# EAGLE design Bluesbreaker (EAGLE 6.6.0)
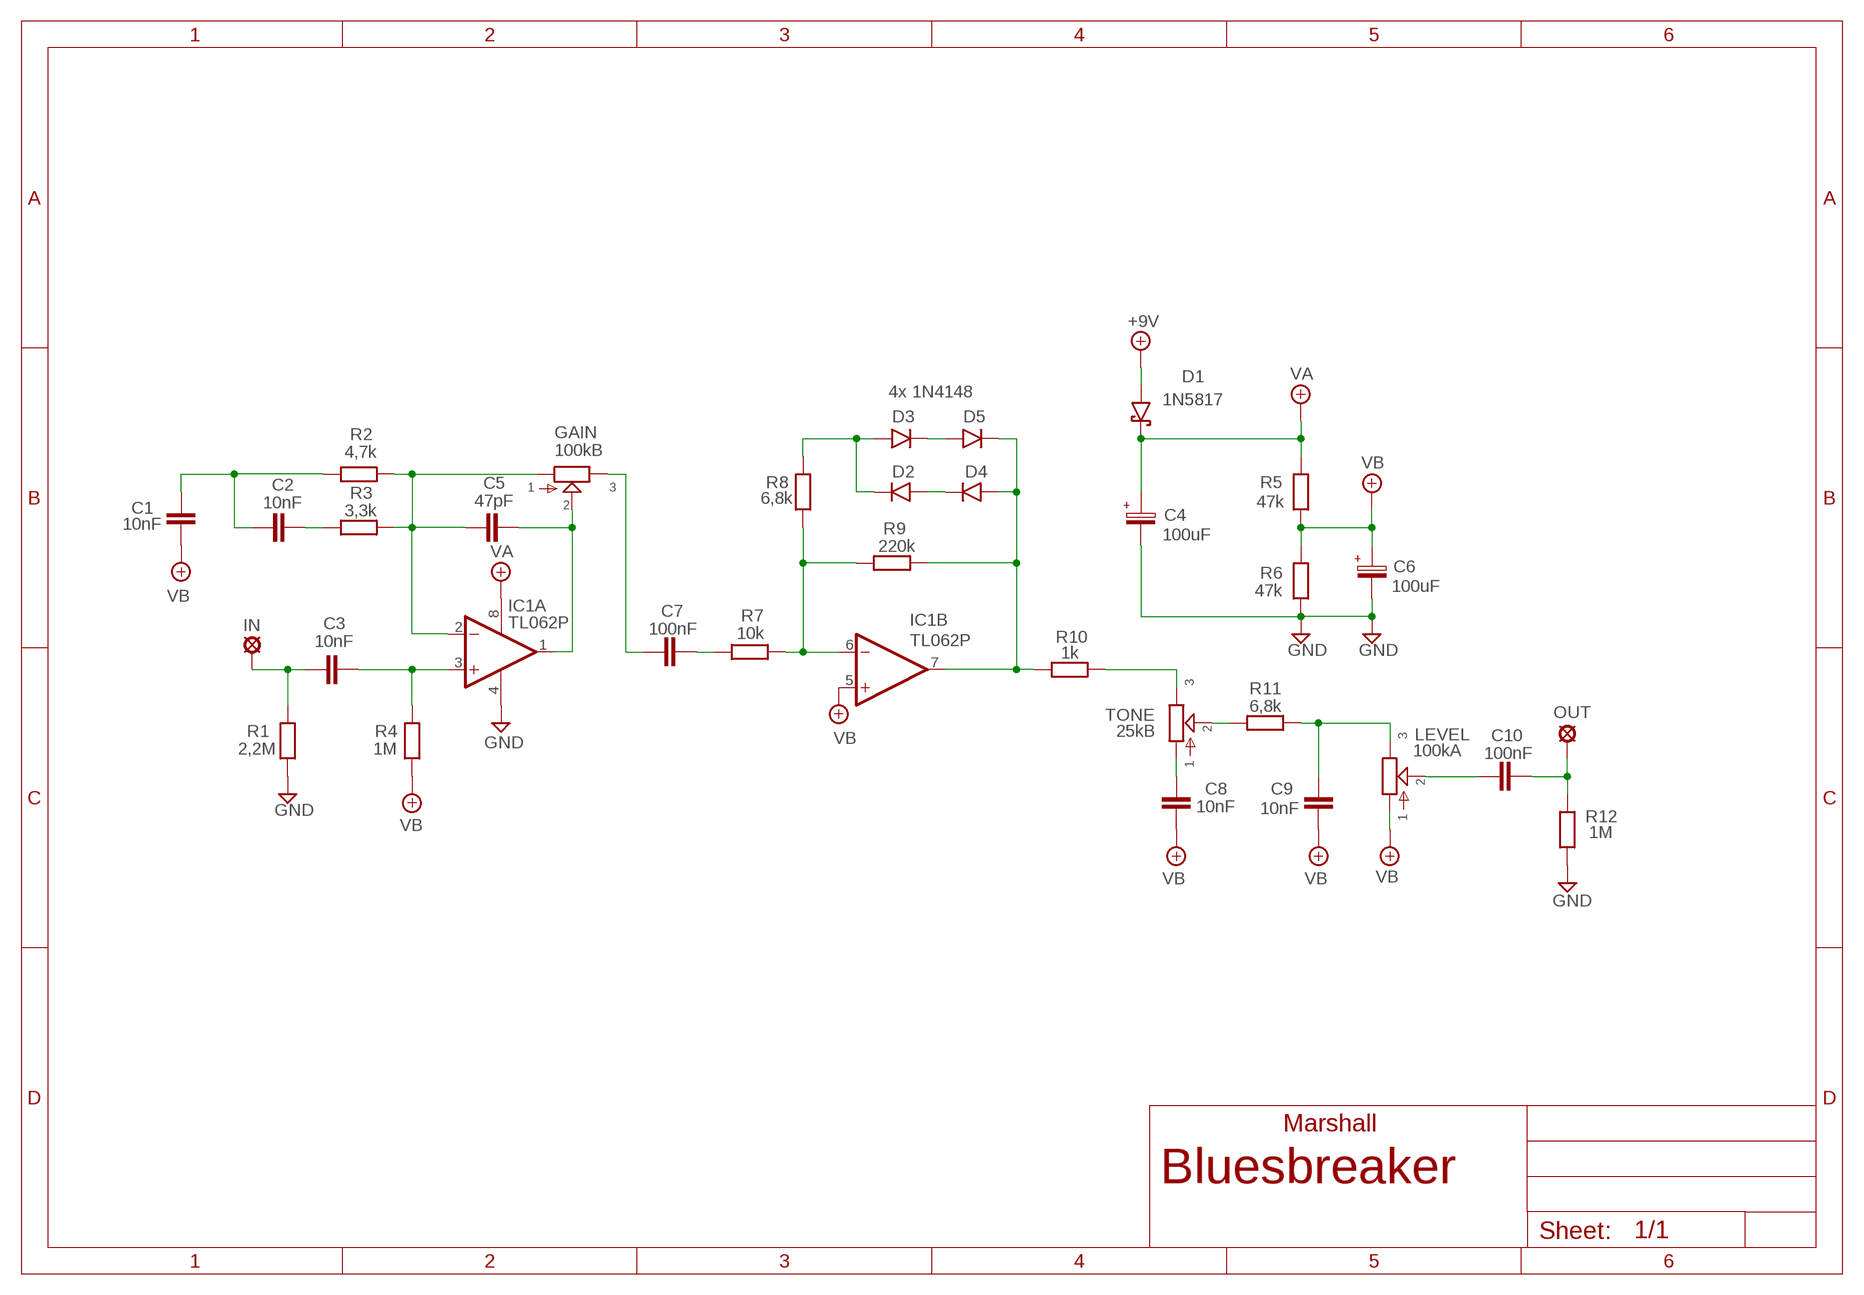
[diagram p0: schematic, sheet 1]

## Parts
+9V  +9V  +9V(T)1  [ROUND]
C1  10nF  1NF-15NF  [3,5MM]
C2  10nF  1NF-15NF  [3,5MM]
C3  10nF  1NF-15NF  [3,5MM]
C4  100uF  063-EU  [063_025]
C5  47pF  050X030_0251  [050X030_025]
C6  100uF  063-EU  [063_025]
C7  100nF  100NF-220NF  [7,5MM]
C8  10nF  1NF-15NF  [3,5MM]
C9  10nF  1NF-15NF  [3,5MM]
C10  100nF  100NF-220NF  [7,5MM]
D1  1N5817  [DO41-3]
D2  1N4148-3  [DO35-3]
D3  4x 1N4148  1N4148-3  [DO35-3]
D4  1N4148-3  [DO35-3]
D5  1N4148-3  [DO35-3]
GAIN  100kB  POT-EU16MM  [16MM]
GND  GND  GND(T)1  [ROUND]
GND5  GND  GND(T)1  [ROUND]
IC1  TL062P  [DIL08]
IN  MCS10B  [MCS10B]
LEVEL  100kA  POT-EU16MM  [16MM]
OUT  MCS10B  [MCS10B]
R1  2,2M  6MM-EU3  [R0207/3]
R2  4,7k  6MM-EU3  [R0207/3]
R3  3,3k  6MM-EU3  [R0207/3]
R4  1M  6MM-EU3  [R0207/3]
R5  47k  6MM-EU3  [R0207/3]
R6  47k  6MM-EU3  [R0207/3]
R7  10k  6MM-EU3  [R0207/3]
R8  6,8k  6MM-EU3  [R0207/3]
R9  220k  6MM-EU3  [R0207/3]
R10  1k  6MM-EU3  [R0207/3]
R11  6,8k  6MM-EU3  [R0207/3]
R12  1M  6MM-EU3  [R0207/3]
TONE  25kB  POT-EU16MM  [16MM]

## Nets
+9V: +9V.1(+9V) D1.A
GND: C4.- C6.- GND5.1(GND) GND.1(GND) IC1.4(P:V-) R1.1 R6.1 R12.2
N$1: C3.2 IN.MP R1.2
N$2: C7.P$1 GAIN.3
N$3: C7.P$2 R7.2
N$4: C3.1 IC1.3(A:+IN) R4.2
N$5: C5.1 GAIN.1 IC1.2(A:-IN) R2.1 R3.1
N$6: C5.2 GAIN.2 IC1.1(A:OUT)
N$7: IC1.6(B:-IN) R7.1 R8.2 R9.2
N$8: C1.1 C2.2 R2.2
N$9: C2.1 R3.2
N$10: R10.1 TONE.3
N$11: D3.C D5.A
N$12: D4.A D5.C IC1.7(B:OUT) R9.1 R10.2
N$13: D2.A D4.C
N$14: C8.1 TONE.1
N$15: D2.C D3.A R8.1
N$16: R11.2 TONE.2
N$17: C9.1 LEVEL.3 R11.1
N$18: C10.P$1 LEVEL.2
N$19: C10.P$2 OUT.MP R12.1
VA: C4.+ D1.C IC1.8(P:V+) R5.2
VB: C1.2 C6.+ C8.2 C9.2 IC1.5(B:+IN) LEVEL.1 R4.1 R5.1 R6.2

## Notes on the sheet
- Marshall

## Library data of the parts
+9V = gm-supply:+9V(T): +9V Voltage Supply
C1-C3 C8 C9 = Mylar Kondensaattorit:1NF-15NF: 1nF-15nF
C4 C6 = Elektrolyytit:063-EU
C5 = Keraamiset kondensaattorit:050X030_025: 47 - 120pF
C7 C10 = Mylar Kondensaattorit:100NF-220NF: 100nF-220nF
D1 = Diodit:1N5817
D2-D5 = Diodit:1N4148: Fast Switching Diode
GAIN LEVEL TONE = gm-pots:POT-EU
GND GND5 = gm-supply:GND(T): Ground
IC1 = Operaatiovahvistimet:TL062: OP AMP
IN OUT = Padit:MCS10B: SOLDER PAD
R1-R12 = Vastukset:6MM-EU: 6mm Resistors (European schematic symbol)

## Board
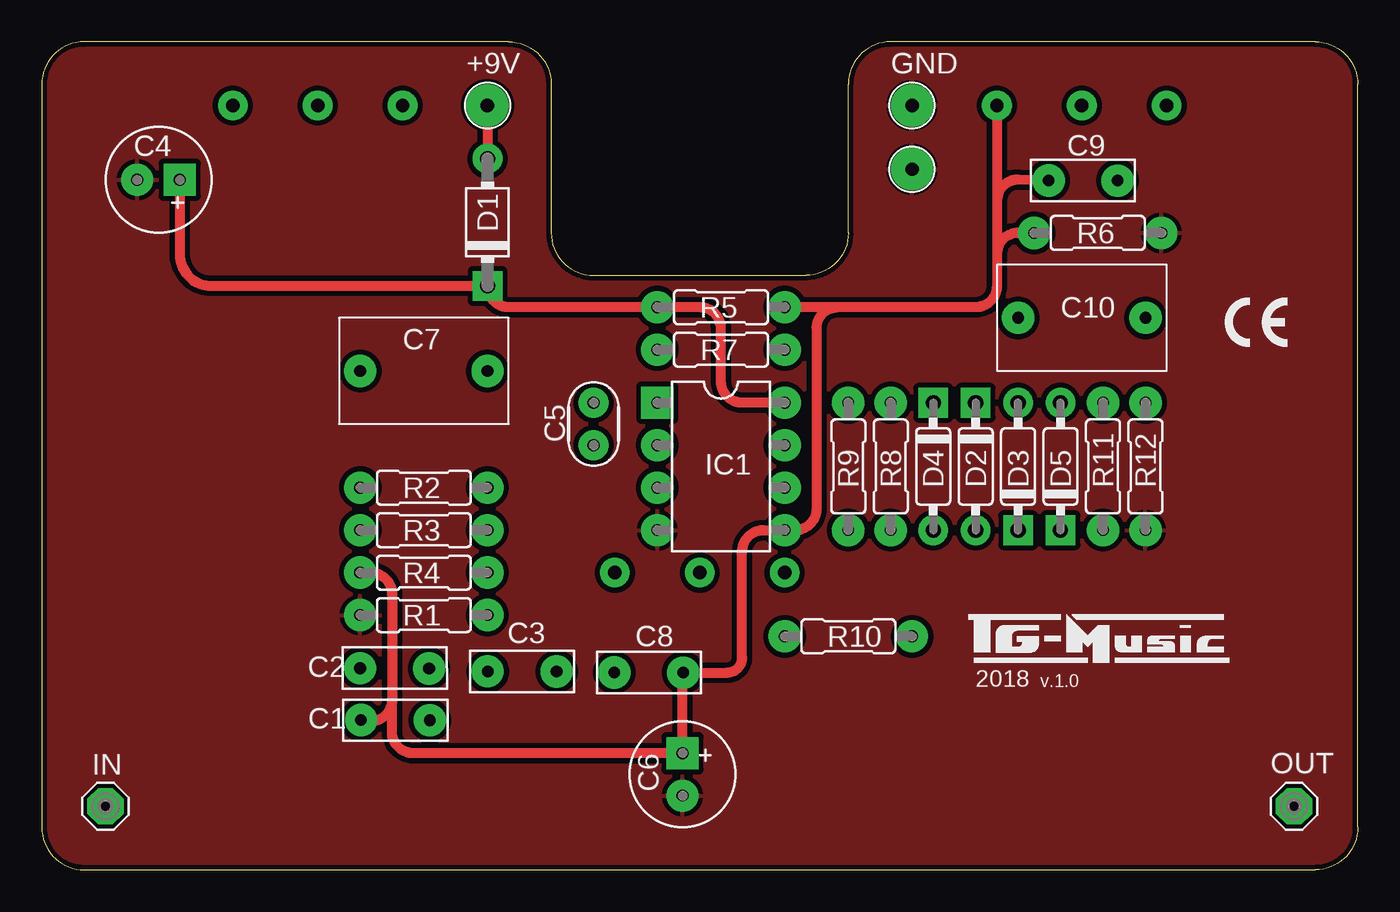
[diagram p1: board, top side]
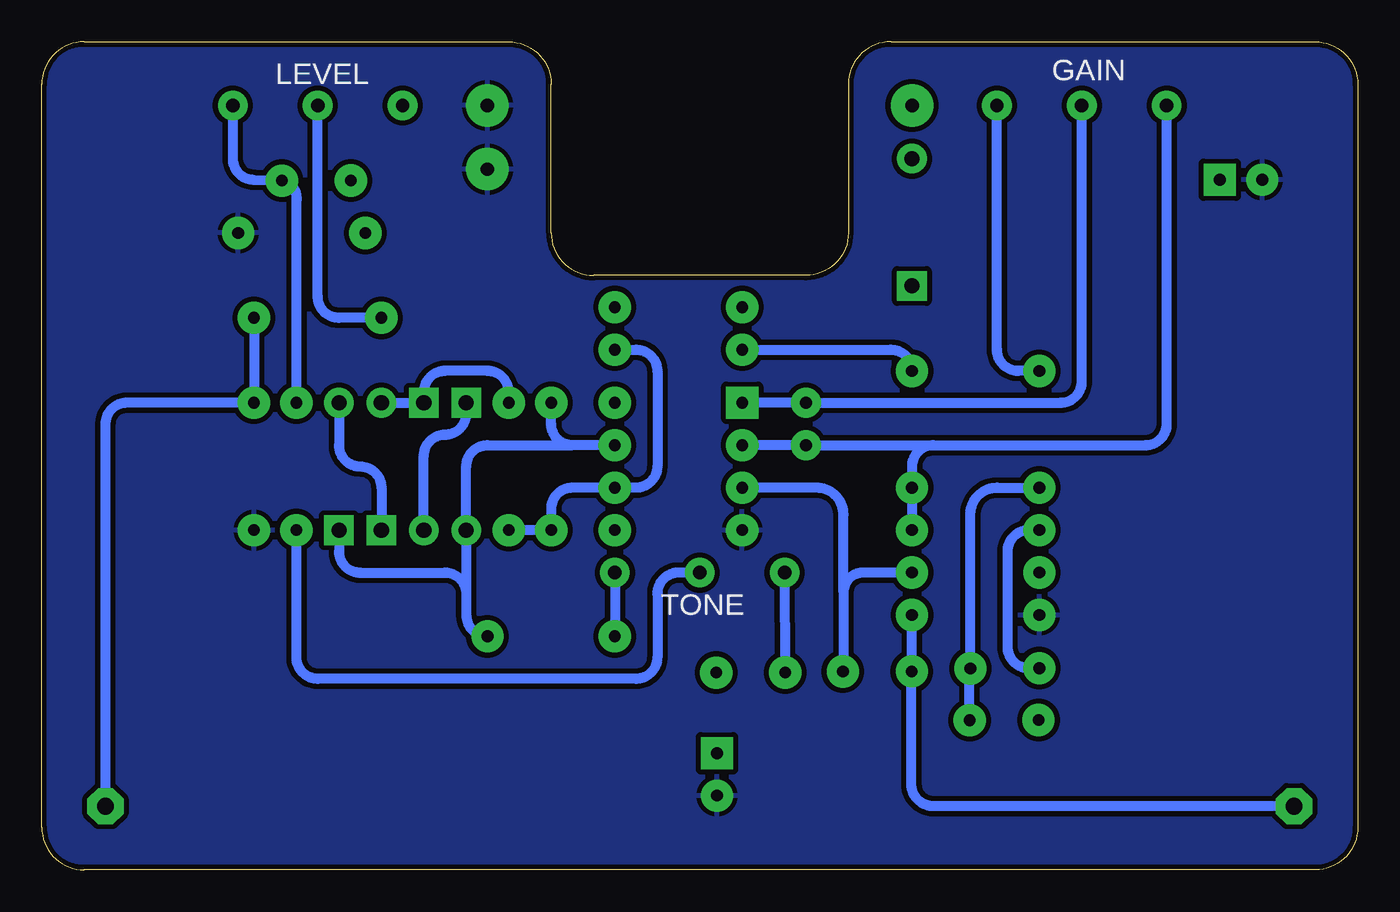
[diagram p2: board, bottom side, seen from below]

Size 78.74 x 49.53 mm. Coordinates in mm from the lower left corner, seen from the top.
Outline: 78.74,2.54 78.74,46.99 arc90 76.2,49.53 50.8,49.53 arc90 48.26,46.99 48.26,38.1 arc-90 45.72,35.56 33.02,35.56 arc-90 30.48,38.1 30.48,46.99 arc90 27.94,49.53 2.54,49.53 arc90 0,46.99 0,2.54 arc90 2.54,0 76.2,0 arc90 78.74,2.54
Copper layers (1*16): Top 0.035mm / dielectric 1.5mm / Bottom 0.035mm
Design rules "ITEADstudio": minimum track width 10mil, minimum drill 12mil, track to track 12mil, track to pad 12mil, pad to pad 12mil, via to via 12mil, smd to smd 0mil, copper to edge 12mil, drill to drill 12mil, minimum pad ring 10mil, minimum via ring 6mil, stop-mask expansion 4mil, vias tented up to drill 100mil, thermal gap 10mil

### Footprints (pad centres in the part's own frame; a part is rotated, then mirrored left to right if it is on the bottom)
ROUND = drill 0.8 pad 2.54: 1 0,0
3,5MM = drill 0.7 pad 1.93: 1 -1.905,0; 2 2.221,-0.016
063_025 = drill 0.7 pad 1.93 square: + -1.27,0 | drill 0.7 pad 1.93: - 1.27,0
050X030_025 = drill 0.7 pad 1.778: 1 -1.27,0; 2 1.27,0
7,5MM = drill 0.7 pad 1.93: P$1 -3.81,0; P$2 3.81,0
DO41-3 = drill 0.9 pad 1.778: A 3.81,0 | drill 0.9 pad 1.778 square: C -3.81,0
DO35-3 = drill 0.9 pad 1.778: A 3.81,0 | drill 0.9 pad 1.778 square: C -3.81,0
16MM = drill 0.8 pad 1.778: 1 5.08,0; 2 0,0; 3 -5.08,0
DIL08 = drill 0.7 pad 1.93 square: 1 -3.81,-3.81 | drill 0.7 pad 1.93: 2 -1.27,-3.81; 3 1.27,-3.81; 4 3.81,-3.81; 5 3.81,3.81; 6 1.27,3.81; 7 -1.27,3.81; 8 -3.81,3.81
MCS10B = drill 1.016 pad 2.159 octagon: MP 0,0
R0207/3 = drill 0.7 pad 1.93: 1 -3.81,0; 2 3.81,0

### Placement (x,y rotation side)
+9V  26.67,45.72 0 top
C1  21.32,8.95 180 top
C2  20.95,12.06 0 top
C3  28.9,11.86 180 top
C4  6.99,41.27 180 top
C5  33.02,26.67 90 top
C6  38.34,5.71 270 top
C7  22.86,29.84 0 top
C8  36.17,11.81 0 top
C9  62.47,41.23 180 top
C10  62.23,33.02 0 top
D1  26.67,38.73 90 top
D2  55.88,24.13 270 top
D3  58.42,24.13 90 top
D4  53.34,24.13 270 top
D5  60.96,24.13 90 top
GAIN  16.51,45.72 0 bottom
GND  52.07,45.72 0 top
GND5  52.07,41.91 0 top
IC1  40.64,24.13 270 top
IN  3.81,3.81 0 top
LEVEL  62.23,45.72 0 bottom
OUT  74.93,3.81 0 top
R1  22.86,15.24 0 top
R2  22.86,22.86 180 top
R3  22.86,20.32 180 top
R4  22.86,17.78 0 top
R5  40.64,33.66 180 top
R6  63.18,38.1 180 top
R7  40.64,31.11 180 top
R8  50.8,24.13 270 top
R9  48.26,24.13 270 top
R10  48.26,13.97 0 top
R11  63.5,24.13 270 top
R12  66.04,24.13 270 top
TONE  39.37,17.78 0 bottom

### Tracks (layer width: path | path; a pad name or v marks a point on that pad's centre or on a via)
+9V
  Top 0.61: +9V.1 D1.A
GND
  pour Bottom: 0,2.54 0,46.99 arc-90 2.54,49.53 27.94,49.53 arc-90 30.48,46.99 30.48,38.1 arc90 33.02,35.56 45.72,35.56 arc90 48.26,38.1 48.26,46.99 arc-90 50.8,49.53 76.2,49.53 arc-90 78.74,46.99 78.74,2.54 arc-90 76.2,0 2.54,0 arc-90
  pour Top: 0,1.91 0,46.99 arc-90 2.54,49.53 27.94,49.53 arc-90 30.48,46.99 30.48,38.1 arc90 33.02,35.56 45.72,35.56 arc90 48.26,38.1 48.26,46.99 arc-90 50.8,49.53 76.2,49.53 arc-90 78.74,46.99 78.74,2.54 arc-90 76.2,0 2.54,0 arc-90
N$1
  Bottom 0.61: IN.MP 25.38,3.81 arc90 26.71,5.14 26.71,11.84 arc90 C3.2 26.68,15.23 arc90 R1.2
N$2
  Bottom 0.61: C7.P$1 20.32,29.84 arc90 21.59,31.11 GAIN.3
N$3
  Bottom 0.61: R7.2 27.94,31.11 arc90 C7.P$2
N$4
  Bottom 0.61: R4.2 29.59,17.78 arc-90 30.77,16.61 | 30.77,16.61 30.77,11.9 arc90 C3.1 | 30.77,16.61 30.77,21.24 arc-90 32.38,22.86 IC1.3
N$5
  Bottom 0.61: R3.1 R2.1 26.67,24.13 arc90 25.4,25.4 | IC1.2 C5.1 25.4,25.4 | GAIN.1 11.43,26.67 arc90 12.7,25.4 25.4,25.4
N$6
  Bottom 0.61: IC1.1 C5.2 17.78,27.94 arc-90 16.51,29.21 GAIN.2
N$7
  Bottom 0.61: R8.2 R9.2 48.26,21.59 arc90 46.99,22.86 45.09,22.86 IC1.6 43.18,22.86 arc-90 41.91,24.13 41.91,29.84 arc-90 43.18,31.11 R7.1
N$8
  Bottom 0.61: C1.1 23.23,12 arc90 C2.2 23.18,21.27 arc90 21.59,22.86 R2.2
N$9
  Bottom 0.61: R3.2 19.68,20.32 arc-90 20.95,19.05 20.95,13.34 arc-90 19.68,12.06 C2.1
N$10
  Bottom 0.61: TONE.3 R10.1
N$11
  Bottom 0.61: D5.A 60.96,25.4 arc-90 59.69,24.13 arc90 58.42,22.86 D3.C
N$12
  Bottom 0.61: IC1.7 46.99,25.4 | 46.99,25.4 arc90 48.26,26.67 R9.1 | 46.99,25.4 52.07,25.4 arc-90 53.34,24.13 D4.A 53.34,16.51 | 53.34,16.51 53.34,15.24 arc-90 R10.2 | D5.C 60.96,19.05 arc-90 59.69,17.78 54.61,17.78 arc90 53.34,16.51
N$13
  Bottom 0.61: D2.A 55.88,24.77 arc90 54.61,26.04 arc-90 53.34,27.3 D4.C
N$14
  Bottom 0.61: TONE.1 C8.1
N$15
  Bottom 0.61: D3.A D2.C 55.88,28.57 arc90 54.61,29.84 52.07,29.84 arc90 50.8,28.57 R8.1
N$16
  Bottom 0.61: TONE.2 40.64,17.78 arc-90 41.91,16.51 41.91,12.7 arc90 43.18,11.43 62.23,11.43 arc90 63.5,12.7 R11.2
N$17
  Bottom 0.61: LEVEL.3 67.31,42.55 arc-90 66.04,41.27 C9.1 arc90 63.5,40.01 R11.1
N$18
  Bottom 0.61: C10.P$1 60.96,33.02 arc90 62.23,34.29 LEVEL.2
N$19
  Bottom 0.61: C10.P$2 R12.1 73.66,27.94 arc-90 74.93,26.67 OUT.MP
VA
  Top 0.61: IC1.8 41.91,27.94 arc-90 40.64,29.21 40.64,32.38 arc90 39.37,33.66 R5.2 27.94,33.66 arc-90 D1.C 10.16,34.92 arc-90 8.26,36.83 C4.+
VB
  Top 0.61: LEVEL.1 57.15,40.01 | 57.15,40.01 57.15,36.83 | 57.15,36.83 57.15,34.92 arc-90 55.88,33.66 47.62,33.66 | 47.62,33.66 R5.1 | 47.62,33.66 arc90 46.35,32.38 46.35,21.59 arc-90 45.09,20.32 IC1.5 43.18,20.32 arc90 41.91,19.05 41.91,12.7 arc-90 41.01,11.8 C8.2 arc90 38.34,11.75 C6.+ 22.23,6.98 arc-90 20.95,8.26 20.95,10.16 | R4.1 19.68,17.78 arc-90 20.95,16.51 20.95,10.16 | 20.95,10.16 arc-90 19.68,8.89 19.18,8.89 arc-90 C1.2 | R6.2 58.42,38.1 arc90 57.15,36.83 | C9.2 58.44,41.29 arc90 57.15,40.01

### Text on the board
tNames: 2018 | v.1.0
